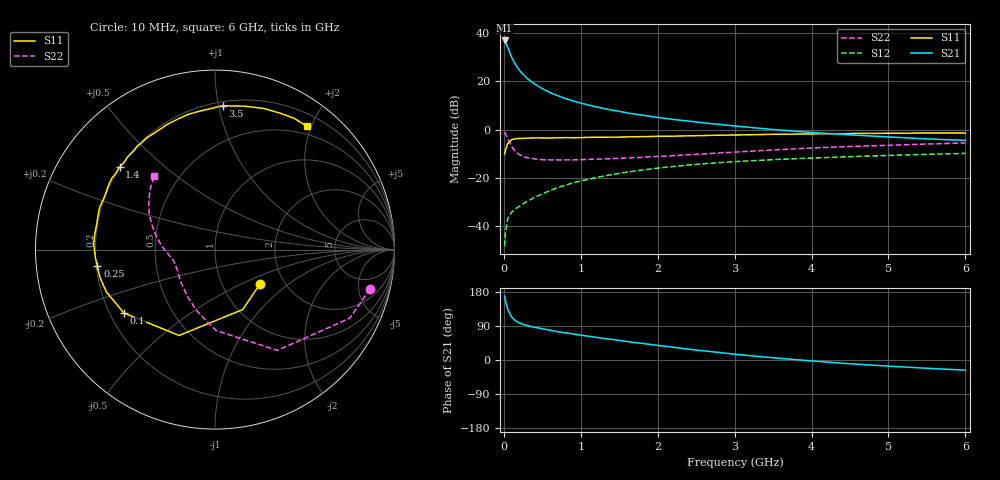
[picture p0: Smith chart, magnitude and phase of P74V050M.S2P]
! SIEMENS Small Signal Semiconductors
! BFP196
! Si NPN RF Bipolar Junction Transistor in SOT143
! VCE = 4 V  IC = 50 mA
! Common Emitter S-Parameters:  May  1996
# GHz  S  MA  R  50
!  f  S11  S21  S12  S22
! GHz  MAG  ANG  MAG  ANG  MAG  ANG  MAG  ANG
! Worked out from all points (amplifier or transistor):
!   36 points, 10 MHz to 6 GHz, reference 50 ohm
!   highest |S21| = 36.9 dB at 10 MHz (marker M1)
!   |S21| within 3 dB of that: start of sweep to 51.59 MHz
!   unconditionally stable (mu >= 1): 458.4 MHz to 4.344 GHz
!   at 250 MHz: K = 0.84, MSG = 26.8 dB, |S12| = -30.7 dB
!   at 1.4 GHz: K = 1.08, MAG = 11.6 dB, |S12| = -18.6 dB
!   at 6 GHz: K = 0.98, MSG = 2.7 dB, |S12| = -9.8 dB
!   S11 on the Smith chart (normalised r, x): 10 MHz: 1.51, -0.64; 100 MHz: 0.26, -0.30; 250 MHz: 0.20, -0.07; 1.4 GHz: 0.20, +0.36; 3.5 GHz: 0.23, +1.03; 6 GHz: 0.37, +1.93
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0.01  0.3155 -37.1  69.98 168.5  0.0039 79.6  0.8916 -14.2
0.02  0.3679 -65.1  65.34 157.2  0.0072 72.6  0.8426 -27.0
0.05  0.5185 -112.7  50.27 133.7  0.0144 56.4  0.6601 -58.3
0.1  0.6182 -145.1  31.8 113.8  0.0195 48.1  0.4507 -89.2
0.15  0.649 -158.6  22.41 104.0  0.0228 48.7  0.3548 -106.9
0.2  0.6595 -166.3  17.21 98.0  0.0259 51.1  0.3065 -119.2
0.25  0.6617 -172.1  13.84 94.0  0.0292 53.4  0.279 -128.6
0.3  0.6678 -176.1  11.61 91.1  0.0327 56.6  0.2648 -134.9
0.4  0.6769 177.2  8.787 86.4  0.0399 59.0  0.2477 -144.6
0.5  0.6752 172.4  7.042 82.4  0.0472 60.9  0.2397 -150.9
0.6  0.6738 167.7  5.874 78.5  0.0552 61.9  0.2373 -155.4
0.7  0.6793 163.4  5.055 74.7  0.0633 62.6  0.2371 -158.7
0.9  0.6818 156.1  3.93 68.7  0.0795 61.4  0.2374 -163.7
1.1  0.693 149.0  3.234 62.7  0.0946 59.9  0.2431 -167.1
1.4  0.7026 139.1  2.547 54.4  0.1173 56.4  0.2516 -171.2
1.7  0.7122 129.5  2.103 46.0  0.1391 52.4  0.2643 -175.6
2.2  0.7335 116.4  1.629 33.7  0.173 45.2  0.2897 177.9
3  0.7749 96.9  1.193 15.2  0.2184 33.5  0.3433 165.5
3.5  0.8024 87.0  1.008 5.9  0.2399 26.6  0.3809 158.0
4.5  0.8321 70.9  0.782 -9.9  0.277 14.7  0.4492 145.2
5.5  0.8546 58.9  0.645 -21.8  0.3092 4.0  0.5051 134.7
6  0.8563 53.4  0.601 -26.8  0.3241 -1.7  0.5303 129.5
